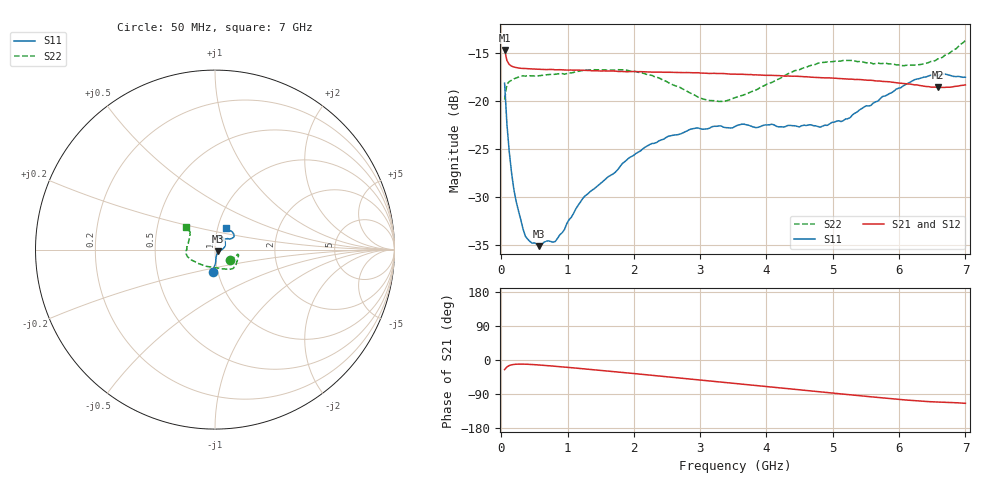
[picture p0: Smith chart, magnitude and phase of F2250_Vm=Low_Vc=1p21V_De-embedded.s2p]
! Integrated Device Technology
! Corporate Headquarters
! 6024 Silver Creek Valley Road
! San Jose, CA 95138  USA
! Phone:  1-408-284-8200
! Toll Free:  1-800-223-1366
! Webpage:  http://www.idt.com/
! Timing and RF Division
! 515 Groton Road, Suite 102
! Westford, MA 01886-6024
! Device:  F2250
! Description: Voltage Variable RF Attenuator
! Frequency:  50.0 -  6000.00 MHz
! Package:  3x3 mm Thin QFN Plastic Package: 16 pin
! Ports:  2 RF, 3 DC
!  Pin  1  = GND
!  Pin  2  = NC
!  Pin  3  = RF1  = Port 1
!  Pin  4  = NC
!  Pin  5  = GND
!  Pin  6  = GND
!  Pin  7  = GND
!  Pin  8  = GND
!  Pin  9  = NC
!  Pin 10  = RF2  = Port 2
!  Pin 11  = NC
!  Pin 12  = GND
!  Pin 13  = GND
!  Pin 14  = VCNTRL
!  Pin 15  = VDD
!  Pin 16  = VMODE
! Vcntrl:  1.210 Volts
! Vmode:  +0.000 Volts
! Vdd:  +3.30  Volts
! Current:  1.193 mA
! Data:  The device was measured on a the F2250 evaluation board which has
!  individual transmission lines to the RF pins.  Data was collected
!  using a calibrated network analyzer.  The evaluation board was
!  de-embedded using a TRL calibration technique.
!  The reference plane is the edge of the package pin.
! Misc:  SN 10
!  Action Tracker AT0258
! Date Measured:  2014-11-26
! Date:  2015-10-15  MJV
! Note:
!  Integrated Device Technology supplies this data as a sample of measured
!  data at the package pin for this product.  Your particular data for this
!  product may vary.
!  Data was taken at 25 degrees C.
!  Integrated Device Technology reserves the right to change this data at anytime.
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# GHz S dB R 50
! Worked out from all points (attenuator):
!   201 points, 50 MHz to 7 GHz, reference 50 ohm
!   highest |S21| = -14.66 dB at 50 MHz (marker M1); lowest = -18.6 dB at 6.583 GHz (marker M2)
!   lowest |S11| = -35.1 dB at 571.2 MHz (marker M3), VSWR 1.04, Z = 51.5 - j0.921 ohm
!   |S11| at or under -10 dB: start of sweep to end of sweep
!   |S22| runs from -20.0 to -13.7 dB; largest |S21 - S12| = 0.00048
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0.05  -18.15 -96.4  -14.66 -25.3  -14.66 -25.3  -19.84 -36.1
0.08475  -22.39 -87.7  -15.78 -18.2  -15.80 -18.2  -18.25 -17.7
0.1195  -25.27 -84.5  -16.18 -14.7  -16.18 -14.7  -17.97 -13.1
0.189  -29.19 -76.5  -16.46 -11.7  -16.45 -11.7  -17.69 -11.5
0.22375  -30.47 -70.7  -16.51 -11.1  -16.52 -11.1  -17.60 -11.9
0.36275  -34.10 -53.8  -16.61 -11.0  -16.61 -11.0  -17.40 -13.1
0.57125  -35.14 -30.7  -16.69 -13.2  -16.68 -13.2  -17.36 -18.4
0.6755  -34.62 -28.2  -16.72 -14.6  -16.70 -14.6  -17.27 -21.1
0.8145  -34.65 -19.2  -16.75 -16.6  -16.73 -16.6  -17.21 -25.2
1.2315  -30.14 -8.8  -16.79 -23.1  -16.79 -23.1  -16.80 -35.3
1.9265  -25.93 11.1  -16.94 -34.5  -16.92 -34.5  -16.84 -47.6
2.37825  -24.15 22.5  -16.99 -42.0  -16.96 -42.1  -17.59 -56.9
2.86475  -22.92 38.1  -17.06 -50.4  -17.05 -50.4  -19.22 -74.5
3.07325  -22.92 45.0  -17.10 -54.0  -17.09 -54.0  -19.85 -86.1
3.3165  -22.60 53.7  -17.14 -58.2  -17.12 -58.3  -20.05 -102.2
3.525  -22.66 58.9  -17.20 -61.8  -17.20 -61.8  -19.65 -115.9
4.7065  -22.57 66.0  -17.53 -82.2  -17.51 -82.2  -16.25 -163.1
5.15825  -22.05 50.3  -17.68 -90.1  -17.68 -90.1  -15.77 -172.1
5.85325  -19.23 34.0  -18.00 -101.7  -18.01 -101.8  -16.14 172.7
6.2355  -17.77 34.6  -18.32 -107.4  -18.30 -107.5  -16.25 159.8
6.583  -17.35 42.4  -18.59 -111.0  -18.58 -111.0  -15.61 147.5
7  -17.52 63.3  -18.32 -114.3  -18.32 -114.4  -13.69 142.4
